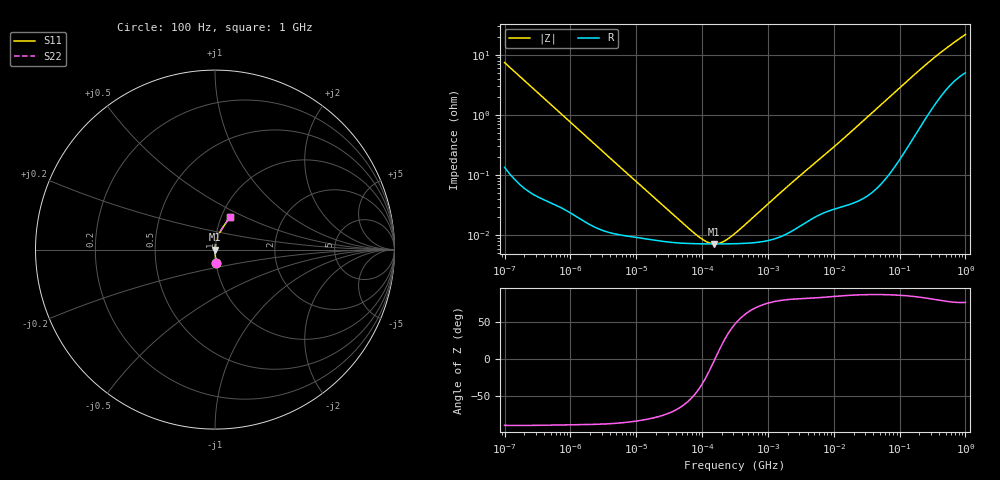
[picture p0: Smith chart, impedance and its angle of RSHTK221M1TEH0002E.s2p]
! RSHTK221M1TEH0002E  S-PARAMETER MODEL  (General Type)
! Model Generated by ELNA Corporation (http://www.ty-top.com)
! Version 1.0
! ELNA Control No. 201215
! Copyright (c) 2020 ELNA CO.,LTD. All Rights Reserved.
! Products Name : CONDUCTIVE POLYMER HYBRID ALUMINUM ELECTROLYTIC CAPACITORS
! Characteristics :
!  Capacitance  :  220uF  ,  Rated voltage  :  25V
!  Operating Temp. Range  :  -55 to +125 degC  ,  Endurance  :  4000hr at 125 degC
!  Dimension D  :  8mm  ,  Dimension L  :  10mm
! Frequency Range : 100Hz - 1GHz
! External Node Assignments :
!  1  o---| |---o  2
# MHz S RI R 50
!Freq[MHz].  S11 Real  S11 Imag  S21 Real  S21 Imag  S12 Real  S12 Imag  S22 Real  S22 Imag
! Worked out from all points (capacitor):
!   401 points, 100 Hz to 1 GHz, reference 50 ohm
!   read as one part in series: C = 215 uF near 108 Hz
!   lowest |Z| = 7.19 mohm at 153.1 kHz (marker M1)
!   series resonance near 156.1 kHz, so ESL is about 4.8 nH
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0.0001  0.00678 -0.0735  0.9932 0.0735  0.9932 0.0735  0.00678 -0.0735
0.000113  0.00541 -0.0652  0.9946 0.0652  0.9946 0.0652  0.00541 -0.0652
0.000183  0.00228 -0.0404  0.9977 0.0404  0.9977 0.0404  0.00228 -0.0404
0.000309  0.00102 -0.024  0.999 0.024  0.999 0.024  0.00102 -0.024
0.001488  0.000206 -0.0051  0.9998 0.0051  0.9998 0.0051  0.000206 -0.0051
0.022131  8.09e-05 -0.000351  0.9999 0.000351  0.9999 0.000351  8.09e-05 -0.000351
0.060604  7.32e-05 -0.000113  0.9999 0.000113  0.9999 0.000113  7.32e-05 -0.000113
0.080353  7.24e-05 -7.37e-05  0.9999 7.37e-05  0.9999 7.37e-05  7.24e-05 -7.37e-05
0.090678  7.22e-05 -5.89e-05  0.9999 5.89e-05  0.9999 5.89e-05  7.22e-05 -5.89e-05
0.153109  7.19e-05 -1.98e-06  0.9999 1.98e-06  0.9999 1.98e-06  7.19e-05 -1.98e-06
0.269153  7.22e-05 5.92e-05  0.9999 -5.92e-05  0.9999 -5.92e-05  7.22e-05 5.92e-05
0.291743  7.23e-05 6.9e-05  0.9999 -6.9e-05  0.9999 -6.9e-05  7.23e-05 6.9e-05
0.316228  7.25e-05 7.92e-05  0.9999 -7.92e-05  0.9999 -7.92e-05  7.25e-05 7.92e-05
1.862087  0.000104 0.0006  0.9999 -0.0006  0.9999 -0.0006  0.000104 0.0006
4.704354  0.000191 0.00144  0.9998 -0.00144  0.9998 -0.00144  0.000191 0.00144
13.96368  0.000318 0.00401  0.9997 -0.00401  0.9997 -0.00401  0.000318 0.00401
69.9842  0.00142 0.0197  0.9986 -0.0197  0.9986 -0.0197  0.00142 0.0197
156.6751  0.00573 0.0431  0.9943 -0.0431  0.9943 -0.0431  0.00573 0.0431
323.5937  0.0202 0.0826  0.9798 -0.0826  0.9798 -0.0826  0.0202 0.0826
568.8529  0.0458 0.1266  0.9542 -0.1266  0.9542 -0.1266  0.0458 0.1266
922.5714  0.0782 0.1746  0.9218 -0.1746  0.9218 -0.1746  0.0782 0.1746
1000  0.0846 0.1841  0.9154 -0.1841  0.9154 -0.1841  0.0846 0.1841
